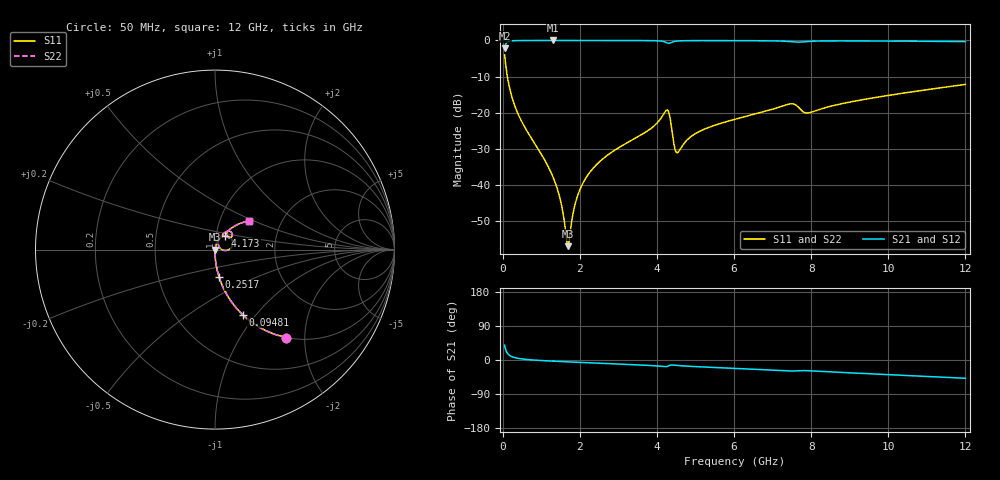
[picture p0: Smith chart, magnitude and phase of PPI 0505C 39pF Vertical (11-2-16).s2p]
# GHz S MA R 50
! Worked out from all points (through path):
!   1601 points, 50 MHz to 12 GHz, reference 50 ohm
!   highest |S21| = -0.01 dB at 1.305 GHz (marker M1); lowest = -2.2 dB at 50 MHz (marker M2)
!   group delay of S21, straight-line fit = 11.9 ps
!   lowest |S11| = -57.0 dB at 1.693 GHz (marker M3), VSWR 1.00, Z = 50.1 - j0.00945 ohm
!   |S11| at or under -10 dB: 121.5 MHz to end of sweep
!   |S22| runs from -57.0 to -4.0 dB; largest |S21 - S12| = 0
!   S11 on the Smith chart (normalised r, x): 50 MHz: 1.00, -1.62; 94.81 MHz: 1.00, -0.85; 251.7 MHz: 1.00, -0.32; 4.173 GHz: 1.11, +0.17; 12 GHz: 1.37, +0.47
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0.05  0.6309 -51.0  0.7756 39.0  0.7756 39.0  0.6309 -51.0
0.0948125  0.3933 -67.1  0.919 22.9  0.919 22.9  0.3933 -67.1
0.2516563  0.1562 -81.5  0.9871 8.3  0.9871 8.3  0.1562 -81.5
0.498125  0.07454 -86.5  0.9963 2.8  0.9963 2.8  0.07454 -86.5
1.30475  0.0129 -87.5  0.9986 -3.1  0.9986 -3.1  0.0129 -87.5
1.491469  0.006356 -81.8  0.9985 -4.0  0.9985 -4.0  0.006356 -81.8
1.648313  0.001909 -47.5  0.9985 -4.7  0.9985 -4.7  0.001909 -47.5
1.693125  0.001421 -3.8  0.9985 -4.9  0.9985 -4.9  0.001421 -3.8
1.879844  0.005454 68.3  0.9984 -5.8  0.9984 -5.8  0.005454 68.3
2.044156  0.009657 74.2  0.9983 -6.5  0.9983 -6.5  0.009657 74.2
2.589375  0.02276 76.6  0.9978 -8.9  0.9978 -8.9  0.02276 76.6
4.038312  0.07539 65.3  0.9856 -16.0  0.9856 -16.0  0.07539 65.3
4.17275  0.09545 53.9  0.9649 -17.3  0.9649 -17.3  0.09545 53.9
4.299719  0.1036 17.8  0.9118 -15.8  0.9118 -15.8  0.1036 17.8
4.456563  0.03337 6.6  0.9683 -13.6  0.9683 -13.6  0.03337 6.6
4.53125  0.02794 34.3  0.981 -14.4  0.981 -14.4  0.02794 34.3
5.031656  0.0525 67.2  0.9936 -17.6  0.9936 -17.6  0.0525 67.2
6.025  0.08108 65.3  0.9926 -22.1  0.9926 -22.1  0.08108 65.3
7.466469  0.1324 48.4  0.9622 -28.9  0.9622 -28.9  0.1324 48.4
8.019156  0.1021 50.6  0.9758 -28.8  0.9758 -28.8  0.1021 50.6
10.01331  0.1736 49.8  0.9793 -38.6  0.9793 -38.6  0.1736 49.8
12  0.246 40.5  0.9633 -48.2  0.9633 -48.2  0.246 40.5
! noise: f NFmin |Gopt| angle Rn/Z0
0.05  0.0004323  0.8775  0.5462  0.0007625
1.372  0.004243  0.6908  4.052  0.002668
2.701  0.007193  0.6501  7.745  0.003889
4.031  0.02096  0.8046  11.63  0.02205
5.36  0.01456  0.6577  15.22  0.007979
6.682  0.0184  0.663  18.81  0.01018
8.012  0.03911  0.7958  22.89  0.03807
9.341  0.02253  0.6281  25.77  0.01082
10.67  0.02336  0.6007  28.86  0.01015
12  0.02563  0.5958  31.97  0.01083
